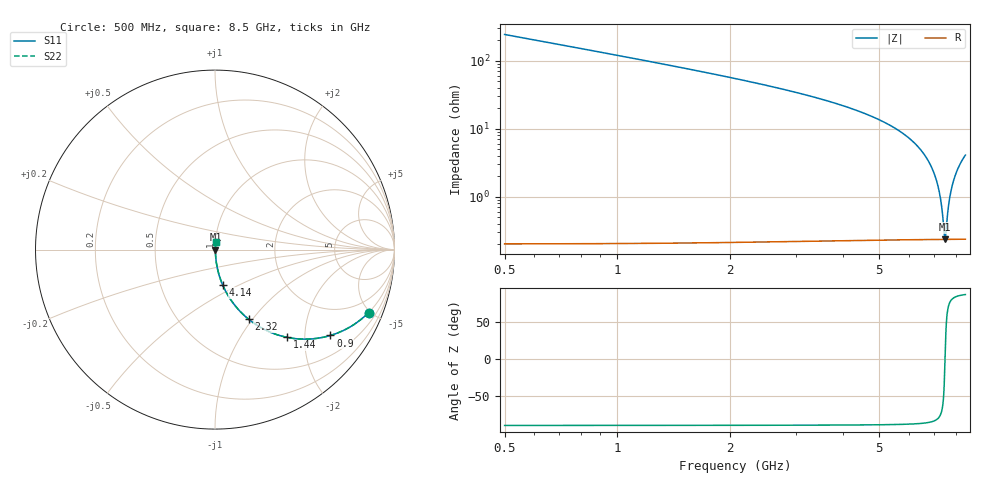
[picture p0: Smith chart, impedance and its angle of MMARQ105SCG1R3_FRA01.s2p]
! MMARQ105SCG1R3_FRA01  S-PARAMETER MODEL  ( General Type )
! Model Generated by TAIYO YUDEN Corporation (http://www.ty-top.com)
! Version 1.0
! TAIYO YUDEN Control No. 200326
! Copyright(c) 2020 TAIYO YUDEN CO.,LTD. All Rights Reserved.
! Product Description (link to TY-COMPAS)
! https://ds.yuden.co.jp/TYCOMPAS/or/detail?pn=MMARQ105SCG1R3BFRA01&u=M
! Products Name : Multilayer Ceramic Capacitors
! Characteristics :
!  Capacitance : 1.3 pF , Rated Voltage : 250V , TCC : CG / C0G
!  Case Size : 1.0 x 0.5 / 0.039 x 0.02 [mm/inch] , Thickness : 0.5 / 0.02 [mm/inch]
!  (Conditions: Temperature = 25 degC , DC Bias Current/Voltage = 0A / 0V)
! External Node Assignments :
!  1  o---| |---o  2
! GND o---------o GND
! Frequency Range : 500MHz  -  8.5GHz  [ 401 STEP ]
# MHz S RI R 50
! Freq[MHz].  S11 Real  S11 Imag  S21 Real  S21 Imag  S12 Real  S12 Imag  S22 Real  S22 Imag
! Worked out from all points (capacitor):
!   401 points, 500 MHz to 8.5 GHz, reference 50 ohm
!   read as one part in series: C = 1.3 pF near 540 MHz
!   lowest |Z| = 236 mohm at 7.5 GHz (marker M1)
!   series resonance near 7.5 GHz, so ESL is about 350 pH
!   S11 on the Smith chart (normalised r, x): 500 MHz: 1.00, -4.88; 900 MHz: 1.00, -2.68; 1.44 GHz: 1.00, -1.64; 2.32 GHz: 1.00, -0.96; 4.14 GHz: 1.00, -0.41; 8.5 GHz: 1.00, +0.08
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500  0.856 -0.3506  0.144 0.3506  0.144 0.3506  0.856 -0.3506
900  0.6428 -0.4784  0.3572 0.4784  0.3572 0.4784  0.6428 -0.4784
1440  0.4021 -0.4891  0.5979 0.4891  0.5979 0.4891  0.4021 -0.4891
1840  0.2821 -0.4484  0.7179 0.4484  0.7179 0.4484  0.2821 -0.4484
2320  0.1868 -0.3875  0.8132 0.3875  0.8132 0.3875  0.1868 -0.3875
3180  0.0924 -0.2862  0.9076 0.2862  0.9076 0.2862  0.0924 -0.2862
4140  0.0426 -0.1965  0.9574 0.1965  0.9574 0.1965  0.0426 -0.1965
4500  0.0315 -0.1683  0.9685 0.1683  0.9685 0.1683  0.0315 -0.1683
5840  0.00905 -0.0816  0.991 0.0816  0.991 0.0816  0.00905 -0.0816
6320  0.00546 -0.0557  0.9945 0.0557  0.9945 0.0557  0.00546 -0.0557
6680  0.00377 -0.0377  0.9962 0.0377  0.9962 0.0377  0.00377 -0.0377
6960  0.00294 -0.0243  0.9971 0.0243  0.9971 0.0243  0.00294 -0.0243
7180  0.00255 -0.0142  0.9974 0.0142  0.9974 0.0142  0.00255 -0.0142
7320  0.00242 -0.0079  0.9976 0.0079  0.9976 0.0079  0.00242 -0.0079
7460  0.00236 -0.00174  0.9976 0.00174  0.9976 0.00174  0.00236 -0.00174
7500  0.00236 -1.79e-06  0.9976 1.79e-06  0.9976 1.79e-06  0.00236 -1.79e-06
7540  0.00236 0.00173  0.9976 -0.00173  0.9976 -0.00173  0.00236 0.00173
7620  0.00239 0.00516  0.9976 -0.00516  0.9976 -0.00516  0.00239 0.00516
7680  0.00242 0.00771  0.9976 -0.00771  0.9976 -0.00771  0.00242 0.00771
7860  0.0026 0.0152  0.9974 -0.0152  0.9974 -0.0152  0.0026 0.0152
8140  0.00308 0.0266  0.9969 -0.0266  0.9969 -0.0266  0.00308 0.0266
8500  0.00404 0.0407  0.996 -0.0407  0.996 -0.0407  0.00404 0.0407
